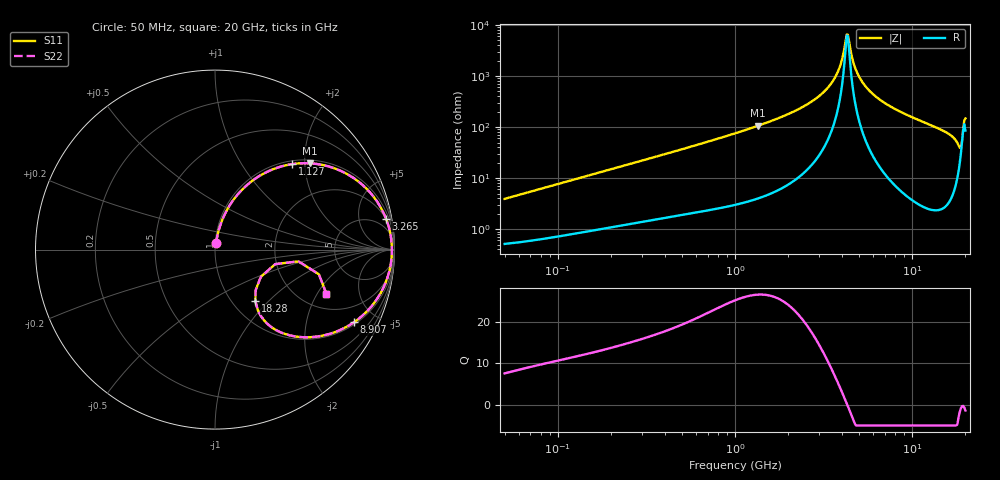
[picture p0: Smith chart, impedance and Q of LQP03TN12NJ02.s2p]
!Murata Part Number: LQP03TN12NJ02
!These Parameters are Measured in Series Mode Connection
!  o--[Z]--o
!Port1  Port2
!  o-------o
!Freq. Start=50[MHz] Stop=20[GHz], 401[Steps]
# Hz S RI R 50
!Freq.(Hz) S11(Real) S11(Imag) S21(Real) S21(Imag) S12(Real) S12(Imag) S22(Real) S22(Imag)
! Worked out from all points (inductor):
!   401 points, 50 MHz to 20 GHz, reference 50 ohm
!   read as one part in series: L = 12.3 nH near 51.52 MHz
!   highest Q = 26.6 at 1.349 GHz (marker M1), where L = 12.5 nH
!   self-resonance near 4.276 GHz
!   S11 on the Smith chart (normalised r, x): 50 MHz: 1.01, +0.08; 1.127 GHz: 1.07, +1.72; 3.265 GHz: 2, +11; 8.907 GHz: 1.10, -3.77; 18.28 GHz: 1.27, -0.84; 20 GHz: 2.71, -2.41
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5e7  0.0066 0.0385  0.9934 -0.0385  0.9934 -0.0385  0.0066 0.0385
1.364002e8  0.0188 0.1004  0.9812 -0.1004  0.9812 -0.1004  0.0188 0.1004
3.721004e8  0.0822 0.2472  0.9178 -0.2472  0.9178 -0.2472  0.0822 0.2472
1e9  0.3679 0.4628  0.6321 -0.4628  0.6321 -0.4628  0.3679 0.4628
1.127304e9  0.4294 0.4761  0.5706 -0.4761  0.5706 -0.4761  0.4294 0.4761
1.349283e9  0.5301 0.4807  0.4699 -0.4807  0.4699 -0.4807  0.5301 0.4807
2.728004e9  0.8992 0.2736  0.1008 -0.2736  0.1008 -0.2736  0.8992 0.2736
3.265178e9  0.9529 0.1724  0.0471 -0.1724  0.0471 -0.1724  0.9529 0.1724
3.792786e9  0.9785 0.0805  0.0215 -0.0805  0.0215 -0.0805  0.9785 0.0805
3.967106e9  0.9825 0.0521  0.0175 -0.0521  0.0175 -0.0521  0.9825 0.0521
4.212059e9  0.9854 0.014  0.0146 -0.014  0.0146 -0.014  0.9854 0.014
4.34015e9  0.9857 -0.00515  0.0143 0.00515  0.0143 0.00515  0.9857 -0.00515
4.748272e9  0.982 -0.0626  0.018 0.0626  0.018 0.0626  0.982 -0.0626
5.194772e9  0.9716 -0.1194  0.0284 0.1194  0.0284 0.1194  0.9716 -0.1194
6.034176e9  0.9392 -0.2107  0.0608 0.2107  0.0608 0.2107  0.9392 -0.2107
7.442007e9  0.8637 -0.3255  0.1363 0.3255  0.1363 0.3255  0.8637 -0.3255
8.907419e9  0.774 -0.405  0.226 0.405  0.226 0.405  0.774 -0.405
1.482269e10  0.4306 -0.4809  0.5694 0.4809  0.5694 0.4809  0.4306 -0.4809
1.696185e10  0.3055 -0.4252  0.6945 0.4252  0.6945 0.4252  0.3055 -0.4252
1.828096e10  0.2253 -0.2882  0.7747 0.2882  0.7747 0.2882  0.2253 -0.2882
1.912117e10  0.3355 -0.0808  0.6645 0.0808  0.6645 0.0808  0.3355 -0.0808
2e10  0.6207 -0.2461  0.3793 0.2461  0.3793 0.2461  0.6207 -0.2461
